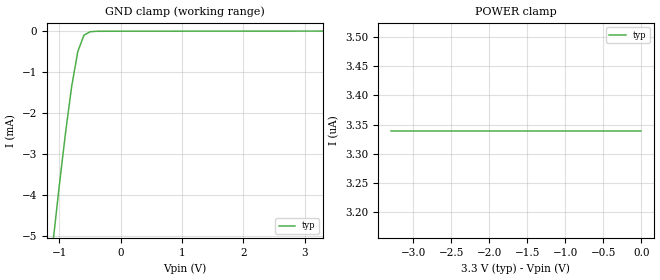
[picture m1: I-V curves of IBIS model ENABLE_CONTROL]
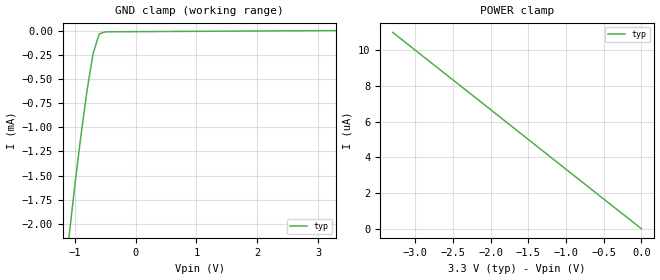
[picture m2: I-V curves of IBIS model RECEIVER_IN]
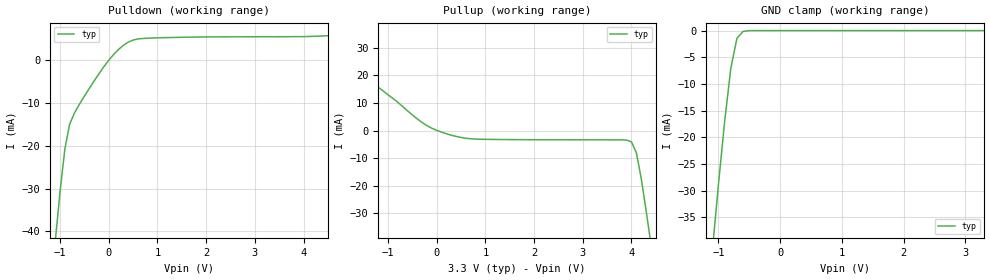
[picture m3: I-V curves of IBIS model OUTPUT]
|   Texas Instruments Incorporated
|   Data Transmissions Products
|   IBIS Model for SN65LVDS116
|   64DGG TSSOP Package
[IBIS Ver]   2.1
[Comment char]   |_char
[File name]   lvds116.ibs
[File Rev]   1.0
[Date]   1Apr99
[Source]   File originated at Texas Instruments Incorporated.
   Data Transmission Products Group.
[Notes]
[Disclaimer]
(C) Copyright Texas Instruments Incorporated 1999
   All rights reserved
  Texas Instruments Incorporated hereby grants the user of this IBIS
model a non-exclusive, nontransferable license to use this IBIS model
under the following terms.  Before using this IBIS model, the user
should read this license.  If the user does not accept these terms,
the IBIS model should be returned to Texas Instruments within 30 days.
  The user is granted this license only to use the IBIS model and
is not granted rights to sell, load, rent, lease or license the IBIS
model in whole or in part, or in modified form to anyone other than
user.  User may modify the IBIS model to suit its specific applications
but rights to derivative works and such modifications shall belong to
Texas Instruments.
  This IBIS model is provided on an "AS IS" basis and Texas Instruments
makes absolutely no warranty with respect to the information contained
herein.  TEXAS INSTRUMENTS DISCLAIMS AND CUSTOMER WAIVES ALL WARRANTIES,
EXPRESS OR IMPLIED, INCLUDING WARRANTIES OF MERCHANTABILITY OR FITNESS
FOR A PARTICULAR PURPOSE. The entire risk as to quality and performance
is with the Customer. ACCORDINGLY, IN NO EVENT SHALL THE COMPANY BE LIABLE
FOR ANY DAMAGES, WHETHER IN CONTRACT OR TORT,INCLUDING ANY LOST PROFITS
OR OTHER INCIDENTAL, CONSEQUENTIAL, EXEMPLARY, OR PUNITIVE DAMAGES ARISING
OUT OF THE USE OR APPLICATION OF THE IBIS model provided in this package.
Further, Texas Instruments reserves the right to discontinue or make changes
without notice to any product herein to improve reliability, function, or
design. Texas Instruments does not convey any license under patent rights
or any other intellectual property rights, including those of third parties.
Contact Texas Instruments at ATTN:DATA TRANSMISSIONS
Thomas Fisher 8505 Forest Lane, M/S 8710, Dallas, TX 75243-4136
[Copyright]   Copyright 1999, Texas Instruments, All Rights Reserved
[Component]   LVDS116DGG
[Manufacturer]  Texas Instruments Incorporated
[Package]
|   typ   min   max
R_pkg   0.068   0.046   0.094
L_pkg   3.798nH   2.565nH   5.991nH
C_pkg   0.564pF   0.297pF   1.022pF
[Pin]   signal_name   model_name   R_pin   L_pin   C_pin
1   GND   GND   0.094   5.991n   0.940p
2   VCC   POWER   0.090   5.514n   1.005p
3   VCC   POWER   0.092   5.261n   0.912p
4   GND   GND   0.092   4.891n   0.805p
5   ENA   ENABLE_CONTROL 0.085   4.561n   0.702p
6   /ENA   ENABLE_CONTROL 0.084   4.247n   0.597p
7   NC   NC
8   NC   NC
9   NC   NC
10   ENB   ENABLE_CONTROL 0.048   3.139n   0.415p
11   /ENB   ENABLE_CONTROL 0.049   3.042n   0.397p
12   NC   NC
13   NC   NC
14   NC   NC
15   GND   GND   0.051   2.589n   0.314p
16   VCC   POWER   0.055   2.604n   0.303p
17   VCC   POWER   0.055   2.597n   0.302p
18   GND   GND   0.052   2.605n   0.315p
19   A   RECEIVER_IN   0.051   2.694n   0.334p
20   B   RECEIVER_IN   0.050   2.772n   0.352p
21   NC   NC
22   /ENC   ENABLE_CONTROL 0.049   2.982n   0.392p
23   ENC   ENABLE_CONTROL 0.049   3.129n   0.413p
24   S0   ENABLE_CONTROL 0.046   3.263n   0.480p
25   S1   ENABLE_CONTROL 0.077   3.592n   0.542p
26   SM   ENABLE_CONTROL 0.081   3.923n   0.557p
27   /END   ENABLE_CONTROL 0.086   4.252n   0.614p
28   END   ENABLE_CONTROL 0.085   4.525n   0.714p
29   GND   GND   0.087   4.810n   0.813p
30   VCC   POWER   0.089   5.135n   0.918p
31   VCC   POWER   0.090   5.486n   1.019p
32   GND   GND   0.090   5.912n   0.936p
33   D4Z   OUTPUT   0.087   5.926n   0.931p
34   D4Y   OUTPUT   0.087   5.496n   1.004p
35   D3Z   OUTPUT   0.087   5.124n   0.902p
36   D3Y   OUTPUT   0.088   4.867n   0.807p
37   D2Z   OUTPUT   0.086   4.514n   0.707p
38   D2Y   OUTPUT   0.085   4.206n   0.605p
39   D1Z   OUTPUT   0.089   3.929n   0.537p
40   D1Y   OUTPUT   0.079   3.584n   0.528p
41   C4Z   OUTPUT   0.048   3.299n   0.481p
42   C4Y   OUTPUT   0.048   3.101n   0.409p
43   C3Z   OUTPUT   0.048   2.969n   0.388p
44   C3Y   OUTPUT   0.048   2.855n   0.369p
45   C2Z   OUTPUT   0.049   2.766n   0.349p
46   C2Y   OUTPUT   0.051   2.696n   0.331p
47   C1Z   OUTPUT   0.052   2.638n   0.315p
48   C1Y   OUTPUT   0.053   2.565n   0.297p
49   B4Z   OUTPUT   0.052   2.574n   0.299p
50   B4Y   OUTPUT   0.051   2.617n   0.313p
51   B3Z   OUTPUT   0.050   2.666n   0.329p
52   B3Y   OUTPUT   0.050   2.769n   0.350p
53   B2Z   OUTPUT   0.049   2.909n   0.378p
54   B2Y   OUTPUT   0.048   2.993n   0.390p
55   B1Z   OUTPUT   0.049   3.176n   0.416p
56   B1Y   OUTPUT   0.048   3.295n   0.483p
57   A4Z   OUTPUT   0.079   3.569n   0.536p
58   A4Y   OUTPUT   0.082   3.908n   0.547p
59   A3Z   OUTPUT   0.086   4.238n   0.613p
60   A3Y   OUTPUT   0.086   4.509n   0.714p
61   A2Z   OUTPUT   0.089   4.863n   0.822p
62   A2Y   OUTPUT   0.090   5.197n   0.923p
63   A1Z   OUTPUT   0.092   5.558n   1.022p
64   A1Y   OUTPUT   0.090   5.947n   0.946p
[Diff_pin]   inv_pin   vdiff   tdelay_typ   tdelay_min   tdelay_max
| The 'xA' pin is Diff_pin and the 'xB' pin is the inv_pin
19   20   0.100   0 0 0
34   33   NA   0 0 0
36   35   NA   0 0 0
38   37   NA   0 0 0
40   39   NA   0 0 0
42   41   NA   0 0 0
44   43   NA   0 0 0
46   45   NA   0 0 0
48   47   NA   0 0 0
50   49   NA   0 0 0
52   51   NA   0 0 0
54   53   NA   0 0 0
56   55   NA   0 0 0
58   57   NA   0 0 0
60   59   NA   0 0 0
62   61   NA   0 0 0
64   63   NA   0 0 0
| Models and submodels in the file (3): ENABLE_CONTROL (Input), RECEIVER_IN (Input), OUTPUT (3-state)
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|   Driver Input / Enable Model
[Model]   ENABLE_CONTROL
Model_type   Input
|Signals   ENA,/ENA,ENB,/ENB,ENC,/ENC,END,/END,S0,S1,SM
Vinh = 2.0
Vinl = 0.8
|   typ   min   max
C_comp   1.0pF   NA   NA
|   typ   min   max
[Temperature Range]   25.0   NA   NA
[Voltage range]   3.3V   3.0V   3.6V
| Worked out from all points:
|   GND clamp passes 1 mA (typ) near -0.76 V on its own axis
[GND_clamp]
|   Voltage   I(typ)   I(min)   I(max)
-3.3V     -43.1mA    NA         NA
-1.1V     -5.08mA    NA         NA
-1V       -3.73mA    NA         NA
-900mV    -2.47mA    NA         NA
-800mV    -1.34mA    NA         NA
-700mV    -493uA     NA         NA
-600mV    -98.5uA    NA         NA
-500mV    -13.3uA    NA         NA
3.3V      3.34uA     NA         NA
[Power_clamp]
| Note that the[POWER_clamp]voltage table is referenced to Vcc
| and is calculated using Vtable=Vcc - Vmeasured.
|   Voltage   I(typ)   I(min)   I(max)
-3.3V     3.34uA     NA         NA
-2.7V     3.34uA     NA         NA
-2V       3.34uA     NA         NA
-800mV    3.34uA     NA         NA
0V        3.34uA     NA         NA
|   Receiver Input MODEL
[Model]   RECEIVER_IN
Model_type   Input
|Signals   A,B
Vinh = 2.0
Vinl = 0.8
|   typ   min   max
C_comp   1.0pF   NA   NA
|   typ   min   max
[Temperature Range]   25.0   NA   NA
[Voltage range]   3.3V   3.0V   3.6V
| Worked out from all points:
|   GND clamp passes 1 mA (typ) near -0.88 V on its own axis
[GND_clamp]
|   Voltage   I(typ)   I(min)   I(max)
-3.3V     -22.5mA    NA         NA
-1.1V     -2.15mA    NA         NA
-1V       -1.59mA    NA         NA
-900mV    -1.08mA    NA         NA
-800mV    -616uA     NA         NA
-700mV    -234uA     NA         NA
-600mV    -34.5uA    NA         NA
-500mV    -13.2uA    NA         NA
-400mV    -12.3uA    NA         NA
3.3V      444pA      NA         NA
[Power_clamp]
| Note that the[POWER_clamp]voltage table is referenced to Vcc
| and is calculated using Vtable=Vcc - Vmeasured.
|   Voltage   I(typ)   I(min)   I(max)
-3.3V     11uA       NA         NA
-2V       6.67uA     NA         NA
-1V       3.33uA     NA         NA
0V        0A         NA         NA
|   Driver Output  MODEL
[Model]   OUTPUT
Model_type   3-state
| Signals   A1Y,A1Z,A2Y,A2Z,A3Y,A3Z,A4Y,A4Z,B1Y,B1Z,B2Y,B2Z,B3Y,B3Z,B4Y,B4Z,
|   C1Y,C1Z,C2Y,C2Z,C3Y,C3Z,C4Y,C4Z,D1Y,D1Z,D2Y,D2Z,D3Y,D3Z,D4Y,D4Z
Vmeas = 1.2V   |Reference voltage for timing measurements
Cref = 5pF   |Timing specification test load capacitance value
Rref = 50   |Note: 50 Ohm load; single ended configuration
Vref = 1.18V   |Timing specification test load voltage
| variable   typ   min   max
C_comp   1.0pF   NA   NA
|   typ   min   max
[Temperature Range]   25.0   NA   NA
[Voltage range]   3.3V   3.0V   3.6V
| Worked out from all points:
|   slope of the pulldown table from 0 to 0.495 V, typ, clamps not added: 105 ohm
|   slope of the pullup table from 0 to 0.495 V, typ, clamps not added: 192 ohm
|   GND clamp passes 1 mA (typ) near -0.67 V on its own axis
[Pulldown]
|   Voltage   I(typ)   I(min)   I(max)
-3.3V     -348mA     NA         NA
-1.1V     -42.6mA    NA         NA
-1V       -30.8mA    NA         NA
-900mV    -20.7mA    NA         NA
-800mV    -14.9mA    NA         NA
-600mV    -10.3mA    NA         NA
-100mV    -1.58mA    NA         NA
200mV     2.42mA     NA         NA
500mV     4.64mA     NA         NA
1.4V      5.26mA     NA         NA
4.1V      5.46mA     NA         NA
6.6V      7.11mA     NA         NA
[Pullup]
|   Voltage   I(typ)   I(min)   I(max)
| Note that the[Pullup]voltage table is referenced to Vcc
| and is calculated using Vtable=Vcc - Vmeasured.
-3.3V     49.3mA     NA         NA
-2.6V     37.7mA     NA         NA
-1.9V     25.6mA     NA         NA
-400mV    4.24mA     NA         NA
200mV     -1.17mA    NA         NA
800mV     -3.11mA    NA         NA
4V        -4.13mA    NA         NA
4.1V      -8.04mA    NA         NA
4.2V      -17.4mA    NA         NA
4.3V      -29mA      NA         NA
4.4V      -41.4mA    NA         NA
6.6V      -348mA     NA         NA
[GND_clamp]
|   Voltage   I(typ)   I(min)   I(max)
| Outputs in High Impedance (off)
-3.3V     -347mA     NA         NA
-1.1V     -41.4mA    NA         NA
-1V       -28.8mA    NA         NA
-900mV    -17.1mA    NA         NA
-800mV    -7.08mA    NA         NA
-700mV    -1.43mA    NA         NA
-600mV    -153uA     NA         NA
-400mV    -866nA     NA         NA
3.3V      -59.7pA    NA         NA
[POWER_clamp]
|   Voltage   I(typ)   I(min)   I(max)
| Note that the [POWER_clamp] voltage table is referenced to Vcc
| and is calculated using Vtable = Vcc - Vmeasured.
| Outputs in Tri-state.
-3.3V     0A         NA         NA
0V        0A         NA         NA
[Ramp]
|   typ   min   max
dV/dt_r   0.346/600ps   NA   NA
dV/dt_f   0.309/600ps   NA   NA
R_load = 100ohm | Note: The measurement is on a differential configuration
